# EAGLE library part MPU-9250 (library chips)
GYRO/ACCEL/COMPASS/9-AXIS
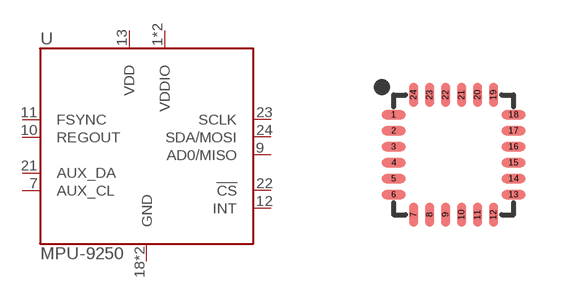
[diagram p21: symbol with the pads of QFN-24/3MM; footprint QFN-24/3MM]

Designator prefix U

## MPU-9250 (DIGIKEY: 1428-1019-1-ND)  [QFN-24/3MM]
1  VDDIO
7  AUX_CL
8  VDDIO
9  AD0/MISO
10  REGOUT
11  FSYNC
12  INT
13  VDD
18  GND
20  GND
21  AUX_DA
22  !CS
23  SCLK
24  SDA/MOSI

## Footprint QFN-24/3MM (pad centres in mm)
smd 0.6 x 0.23: 1 -1.5,1; 2 -1.5,0.6; 3 -1.5,0.2; 4 -1.5,-0.2; 5 -1.5,-0.6; 6 -1.5,-1; 13 1.5,-1; 14 1.5,-0.6; 15 1.5,-0.2; 16 1.5,0.2; 17 1.5,0.6; 18 1.5,1
smd 0.23 x 0.6: 7 -1,-1.5; 8 -0.6,-1.5; 9 -0.2,-1.5; 10 0.2,-1.5; 11 0.6,-1.5; 12 1,-1.5; 19 1,1.5; 20 0.6,1.5; 21 0.2,1.5; 22 -0.2,1.5; 23 -0.6,1.5; 24 -1,1.5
